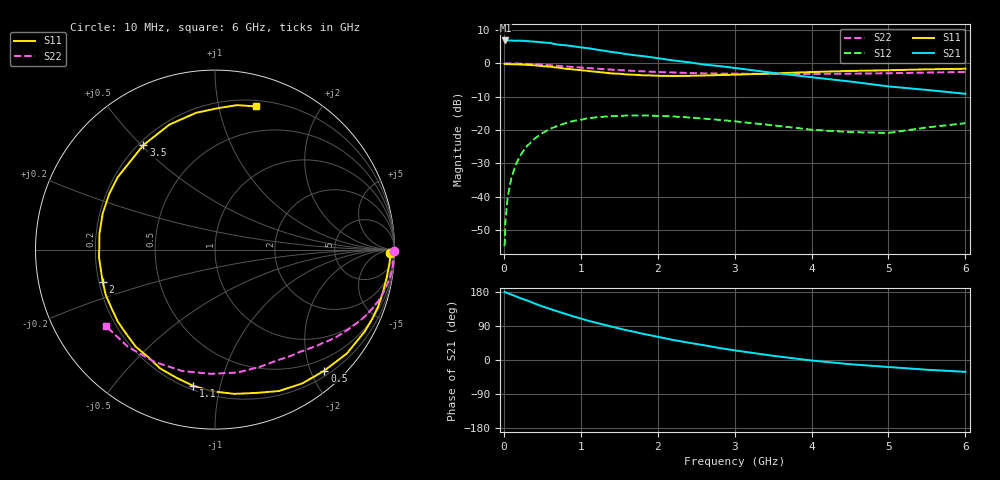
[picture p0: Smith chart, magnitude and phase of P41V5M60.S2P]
! SIEMENS Small Signal Semiconductors
! BFP182
! Si NPN RF Bipolar Junction Transistor in SOT143
! VCE = 1.5 V  IC = 0.6 mA
! Common Emitter S-Parameters:  March  1996
# GHz  S  MA  R  50
!  f  S11  S21  S12  S22
! GHz  MAG  ANG  MAG  ANG  MAG  ANG  MAG  ANG
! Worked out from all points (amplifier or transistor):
!   36 points, 10 MHz to 6 GHz, reference 50 ohm
!   highest |S21| = 6.9 dB at 20 MHz (marker M1)
!   |S21| within 3 dB of that: start of sweep to 1.278 GHz
!   unconditionally stable (mu >= 1): 2.848 GHz to end of sweep
!   at 250 MHz: K = 0.10, MSG = 16.6 dB, |S12| = -26.4 dB
!   at 1.4 GHz: K = 0.51, MSG = 9.7 dB, |S12| = -15.9 dB
!   at 6 GHz: K = 1.22, MAG = 1.6 dB, |S12| = -18.0 dB
!   S11 on the Smith chart (normalised r, x): 10 MHz: 55, -41; 500 MHz: 0.29, -2.22; 1.1 GHz: 0.22, -0.83; 2 GHz: 0.22, -0.13; 3.5 GHz: 0.22, +0.51; 6 GHz: 0.25, +1.30
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0.01  0.9769 -1.0  2.204 179.7  0.0018 88.1  0.9989 -0.3
0.02  0.9791 -1.9  2.208 179.2  0.0041 86.9  0.9999 -0.8
0.05  0.9745 -4.9  2.207 176.2  0.0099 89.5  0.9977 -1.8
0.1  0.9691 -9.5  2.202 172.4  0.0194 83.1  0.9935 -3.6
0.15  0.9651 -14.7  2.183 168.5  0.0292 79.9  0.9947 -5.5
0.3  0.9505 -28.8  2.156 157.4  0.0569 71.4  0.9808 -10.8
0.4  0.9353 -38.2  2.119 149.0  0.0741 65.3  0.9688 -14.2
0.5  0.9089 -47.9  2.066 141.5  0.0895 59.1  0.954 -17.4
0.6  0.8904 -56.8  2.021 134.8  0.1038 53.6  0.9358 -20.5
0.8  0.8313 -73.8  1.871 121.7  0.1262 43.2  0.9005 -26.1
1.1  0.7683 -99.2  1.687 103.5  0.1498 30.0  0.8491 -33.3
1.5  0.6982 -129.3  1.434 83.1  0.1623 15.2  0.7911 -41.4
1.8  0.6624 -150.7  1.289 69.4  0.165 6.8  0.7603 -46.5
2  0.651 -163.9  1.197 61.2  0.1629 1.8  0.7416 -50.0
2.2  0.6475 -175.8  1.106 52.9  0.1594 -3.0  0.7302 -53.6
2.8  0.6666 151.9  0.911 31.8  0.142 -13.0  0.7017 -64.7
3.5  0.7059 124.4  0.72 11.1  0.1174 -17.9  0.6963 -79.8
4  0.7413 110.0  0.62 -1.3  0.101 -14.6  0.6926 -92.0
4.5  0.7693 97.9  0.534 -11.1  0.0928 -8.0  0.7006 -105.1
5  0.788 88.9  0.451 -18.5  0.0903 4.7  0.7104 -118.3
5.5  0.8142 81.3  0.399 -25.7  0.1092 10.8  0.7273 -131.9
6  0.83 73.9  0.349 -31.2  0.1266 12.1  0.7421 -144.9
